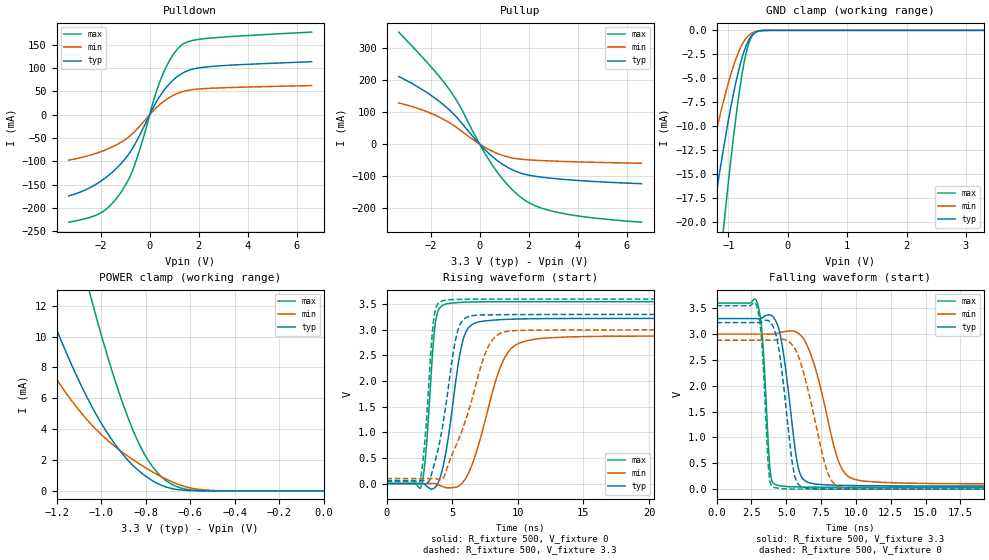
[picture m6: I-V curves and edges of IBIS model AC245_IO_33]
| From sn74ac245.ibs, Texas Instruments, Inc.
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[Model]   AC245_IO_33
Model_type  I/O
Vinl=0.9
Vinh=2.1
Enable   Active-Low
Vref =   0
Rref =   500
Cref =   50p
Vmeas =   1.5
| variable   typ   min   max
C_comp   7.17pF   6.52pF   7.47pF
| C_pullup   12.22pF   7.53pF   17.64pF
| C_pulldown   9.48pF   7.42pF   11.79pF
| C_tri-state   7.17pF   6.52pF   7.47pF
[Temperature Range]   40   100   -40
| Ambient temperature   25   85   -40
[Voltage range]   3.3   3   3.6
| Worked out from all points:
|   slope of the pulldown table from 0 to 0.495 V, typ, clamps not added: 10.8 ohm
|   slope of the pullup table from 0 to 0.495 V, typ, clamps not added: 13.3 ohm
|   GND clamp passes 1 mA (typ) near -0.66 V on its own axis
|   POWER clamp passes 1 mA (typ) near -0.80 V on its own axis
|   rising waveform, R_fixture 500, V_fixture 0: 20-80 % time 1.08ns typ, 1.93ns min, 567ps max; typ from 0 V to 3.22 V
|   falling waveform, R_fixture 500, V_fixture 3.3: 20-80 % time 889ps typ, 1.59ns min, 433ps max; typ from 3.3 V to 0.06 V
|   rising waveform, R_fixture 500, V_fixture 3.3: 20-80 % time 1.18ns typ, 2.17ns min, 579ps max; typ from 0.06 V to 3.3 V
|   falling waveform, R_fixture 500, V_fixture 0: 20-80 % time 824ps typ, 1.5ns min, 413ps max; typ from 3.22 V to 0 V
[GND Clamp]
| AC245_IO_33
|   Voltage   I(typ)   I(min)   I(max)
-3.3V     -138mA     -89.57mA   -186.4mA
-1.545V   -32.5mA    -20.53mA   -51.44mA
-1.525V   -31.52mA   -19.9mA    -50.02mA
-1.285V   -20.46mA   -12.7mA    -33.54mA
-1.1V     -12.96mA   -7.8mA     -21.71mA
-1.07V    -11.84mA   -7.072mA   -19.89mA
-915mV    -6.61mA    -3.72mA    -11.14mA
-780mV    -3.057mA   -1.6mA     -4.922mA
-690mV    -1.428mA   -736uA     -2.066mA
-590mV    -421.2uA   -245.2uA   -490.3uA
-375mV    -8.941uA   -6.826uA   -4.617uA
3.3V      24.75nA    98.15nA    118.6nA
[POWER Clamp]
| AC245_IO_33
|   Voltage   I(typ)   I(min)   I(max)
-3.3V     147mA      100.1mA    236.3mA
-1.42V    19.28mA    12.85mA    37.33mA
-1.28V    13.45mA    9.113mA    27.1mA
-1.245V   12.11mA    8.268mA    24.71mA
-1.06V    5.981mA    4.561mA    13.32mA
-1.04V    5.43mA     4.246mA    12.23mA
-940mV    3.074mA    2.907mA    7.277mA
-850mV    1.557mA    1.958mA    3.706mA
-790mV    852.9uA    1.412mA    2.017mA
-710mV    263.9uA    778.4uA    683.6uA
-520mV    2.489uA    47.32uA    10.24uA
-48.03fV  24.75nA    3.724nA    183.8nA
[Pulldown]
| AC245_IO_33
|   Voltage   I(typ)   I(min)   I(max)
-3.3V     -174mA     -97.37mA   -230.3mA
-1.96V    -141.3mA   -78.58mA   -209.2mA
-1.53V    -123.5mA   -69.07mA   -190.3mA
-1.09V    -100.1mA   -56.34mA   -159.9mA
-805mV    -80.63mA   -45.48mA   -132.8mA
-580mV    -61.18mA   -34.26mA   -103.1mA
195mV     20.15mA    11.19mA    36.58mA
490mV     45.44mA    25.34mA    80.81mA
890mV     70.92mA    39.59mA    123.4mA
1.295V    87.86mA    48.81mA    149mA
2.435V    103.2mA    56.72mA    164.3mA
6.6V      113.8mA    62.59mA    177.3mA
[Pullup]
| AC245_IO_33
|   Voltage   I(typ)   I(min)   I(max)
-3.3V     212mA      128.9mA    351mA
-2.185V   163.3mA    102.7mA    259.8mA
-1.315V   112.8mA    70.92mA    179.3mA
-835mV    75.51mA    46.16mA    123.4mA
-45mV     3.821mA    2.284mA    6.277mA
490mV     -36.97mA   -21.36mA   -62.39mA
1.075V    -69.74mA   -38.49mA   -122.1mA
1.655V    -90.22mA   -47.03mA   -165mA
2.3V      -101.1mA   -50.6mA    -194.1mA
3.22V     -109.1mA   -53.68mA   -214.5mA
4.605V    -116.8mA   -56.81mA   -230.8mA
6.6V      -124mA     -59.91mA   -244.5mA
[Ramp]
| AC245_IO_33
| variable   typ   min   max
dV/dt_r   2.00/1.13E-09   1.78/1.99E-09   2.18/5.87E-10
dV/dt_f   1.99/9.15E-10   1.78/1.63E-09   2.19/4.50E-10
R_load = 500
[Rising Waveform]
| AC245_IO_33
R_fixture =   500
C_fixture =   0
L_fixture =   0
V_fixture =   0
V_fixture_min = 0
V_fixture_max = 0
|   Time   V(typ)   V(min)   V(max)
0s        12.58nV    6.144nV    43.81nV
2.625ns   1.024mV    -156.1uV   -64.39mV
2.995ns   -34.72mV   -198.6uV   599.6mV
3.715ns   -71.56mV   -421.5uV   3.12V
4.505ns   587.5mV    -78.94mV   3.5V
5.535ns   2.45V      -42.39mV   3.534V
6.12ns    2.993V     141.6mV    3.541V
8.76ns    3.199V     2.325V     3.548V
10.5ns    3.213V     2.774V     3.548V
45ns      3.222V     2.882V     3.548V
[Falling Waveform]
| AC245_IO_33
R_fixture =   500
C_fixture =   0
L_fixture =   0
V_fixture =   3.3
V_fixture_min = 3
V_fixture_max = 3.6
|   Time   V(typ)   V(min)   V(max)
0s        3.3V       3V         3.6V
2.94ns    3.299V     3V         3.591V
3.295ns   3.32V      3V         2.937V
3.85ns    3.37V      2.998V     356.9mV
4.35ns    3.195V     3.013V     79.1mV
5.825ns   470.2mV    3.025V     42.97mV
6.69ns    122mV      2.66V      39.49mV
8.745ns   75.71mV    548.5mV    36.64mV
10.02ns   69.02mV    181.7mV    36.03mV
45ns      59.71mV    97.83mV    35.41mV
[Rising Waveform]
| AC245_IO_33
R_fixture =   500
C_fixture =   0
L_fixture =   0
V_fixture =   3.3
V_fixture_min = 3
V_fixture_max = 3.6
|   Time   V(typ)   V(min)   V(max)
0s        59.71mV    97.82mV    35.41mV
2.535ns   60.07mV    97.69mV    22.09mV
2.92ns    44.62mV    97.61mV    830.7mV
3.585ns   328.5mV    99.25mV    3.185V
4.25ns    1.085V     92.03mV    3.564V
5.145ns   2.65V      656.5mV    3.59V
5.655ns   3.13V      967.8mV    3.594V
7.59ns    3.292V     2.582V     3.599V
8.93ns    3.295V     2.955V     3.6V
45ns      3.3V       3V         3.6V
[Falling Waveform]
| AC245_IO_33
R_fixture =   500
C_fixture =   0
L_fixture =   0
V_fixture =   0
V_fixture_min = 0
V_fixture_max = 0
|   Time   V(typ)   V(min)   V(max)
0s        3.222V     2.882V     3.548V
2.89ns    3.221V     2.882V     3.541V
3.245ns   3.234V     2.882V     2.853V
3.75ns    3.257V     2.881V     350.7mV
4.07ns    3.137V     2.881V     39.16mV
5.53ns    358.8mV    2.758V     2.619mV
6.23ns    34.11mV    2.271V     1.256mV
7.915ns   2.465mV    369.5mV    419.8uV
9.015ns   1.361mV    30.9mV     232.7uV
45ns      226.2nV    1.045uV    53.91nV
